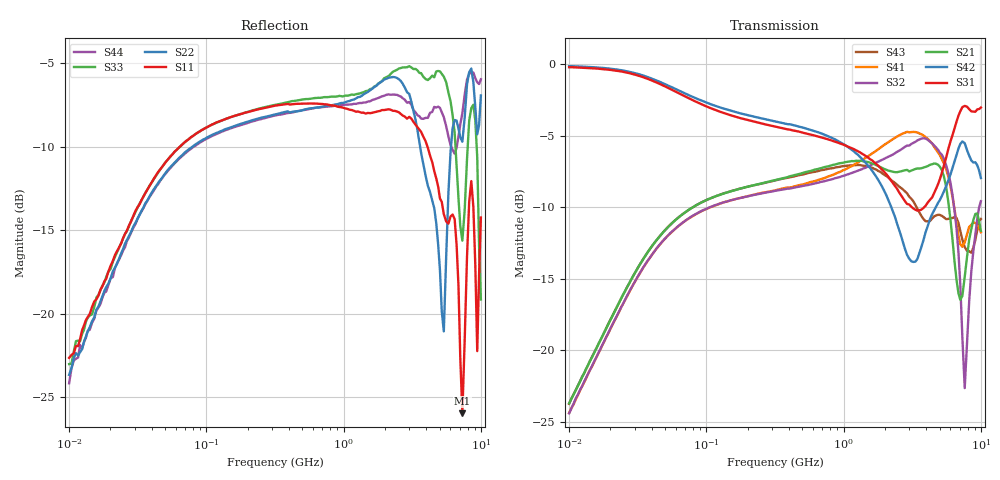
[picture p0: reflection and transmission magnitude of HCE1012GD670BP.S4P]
!Agilent Technologies,E5071C,MY46111244,A.11.31
!Date: Tue May 14 17:32:13 2019
!Data & Calibration Information:
!Freq	S11:SOLT4(ON)	S12:SOLT4(ON)	S13:SOLT4(ON)	S14:SOLT4(ON)
!	S21:SOLT4(ON)	S22:SOLT4(ON)	S23:SOLT4(ON)	S24:SOLT4(ON)
!	S31:SOLT4(ON)	S32:SOLT4(ON)	S33:SOLT4(ON)	S34:SOLT4(ON)
!	S41:SOLT4(ON)	S42:SOLT4(ON)	S43:SOLT4(ON)	S44:SOLT4(ON)
!PortZ  Port1:50+j0  Port2:50+j0  Port3:50+j0  Port4:50+j0
!Above PortZ is port z conversion or system Z0 setting when saving the data.
!When reading, reference impedance value at option line is always used.
# Hz S dB R 50
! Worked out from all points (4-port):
!   201 points, 10 MHz to 10 GHz, reference 50 ohm
!   strongest paths, dB at 10 MHz, 56.66 MHz, 319.3 MHz, 1.79 GHz, 10 GHz:
!     S31: -0.2, -1.8, -4.4, -7.1, -3.0
!     S42: -0.1, -1.6, -4.0, -8.1, -8.0
!     S21: -23.7, -11.1, -8.1, -7.1, -11.7
!     S32: -24.4, -11.7, -8.9, -6.8, -9.6
!     S41: -24.4, -11.7, -8.8, -5.9, -11.8
!     S43: -23.7, -11.1, -8.1, -7.5, -10.8
!   lowest |S11| = -26.0 dB at 7.328 GHz (marker M1), VSWR 1.11, Z = 49.1 - j4.91 ohm
!   |S11| at or under -10 dB: start of sweep to 64.03 MHz; 4.083 GHz to end of sweep
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1e7  -22.66 69.2  -23.74 82.3  -0.21 -4.2  -24.37 -98.2
     -23.71 82.1  -23.67 70.5  -24.38 -98.4  -0.16 -4.0
     -0.22 -4.2  -24.41 -98.1  -23.03 69.7  -23.73 82.1
     -24.39 -98.3  -0.15 -3.9  -23.75 81.9  -24.18 73.8
5.520041e8  -7.40 -0.6  -7.53 8.7  -4.88 -30.5  -8.32 148.5
            -7.51 8.8  -7.72 2.7  -8.45 154.0  -4.56 -31.1
            -4.88 -30.7  -8.45 153.9  -7.14 2.6  -7.66 7.1
            -8.30 149.1  -4.54 -31.3  -7.61 7.1  -7.76 -3.8
3.34031e9  -8.67 -26.9  -7.27 -17.3  -10.19 -176.2  -4.73 5.2
           -7.33 -17.2  -8.37 -49.6  -5.45 19.8  -13.79 136.4
           -10.19 -177.3  -5.43 19.8  -5.33 -19.7  -9.84 -24.5
           -4.75 5.2  -13.80 136.3  -9.86 -24.3  -7.94 -67.3
5.370318e9  -14.04 -81.2  -7.71 -51.3  -7.14 61.1  -6.86 -56.5
            -7.83 -51.3  -21.07 -52.3  -6.64 -52.0  -8.89 11.1
            -7.10 61.4  -6.61 -52.0  -5.80 -88.0  -10.64 -20.2
            -6.93 -56.7  -8.91 10.8  -10.70 -20.2  -8.23 -139.0
7.328245e9  -25.98 -97.2  -16.18 -32.9  -2.95 -11.9  -12.95 -73.3
            -16.21 -33.5  -9.70 -82.4  -19.17 -101.4  -5.41 -39.5
            -3.01 -11.9  -19.07 -102.2  -15.63 -119.4  -12.23 -32.1
            -12.76 -74.3  -5.41 -39.9  -12.28 -31.9  -7.99 160.9
8.515692e9  -12.06 -165.3  -11.42 -39.6  -3.33 -51.3  -11.05 -79.2
            -11.54 -38.8  -5.31 -155.4  -14.58 -35.8  -6.83 -69.5
            -3.30 -51.2  -14.50 -36.3  -7.68 -152.0  -13.18 -29.5
            -11.24 -79.3  -6.73 -69.3  -13.18 -28.6  -5.58 146.5
1e10  -14.24 35.0  -11.77 -101.9  -3.07 -87.2  -11.78 -106.3
      -11.66 -102.7  -6.93 81.7  -9.44 -65.6  -8.00 -93.7
      -3.04 -87.5  -9.58 -65.0  -19.16 177.3  -10.86 -48.9
      -11.76 -106.7  -7.96 -94.4  -10.83 -49.1  -5.96 95.6
